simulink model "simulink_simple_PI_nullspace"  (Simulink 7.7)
settings: Solver=ode23t  StartTime=0.0  StopTime=9.6  RelTol=1e-6
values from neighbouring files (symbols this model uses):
  A = [((-UAfr)/mCpf) (UAfr/mCpf) 0; (UAfr/mCpr) ((-UAro-UAfr)/mCpr) 0; 0 0 0]    [simplemodel.m]
  B = [1/mCpf 0 0 ; 0 1/mCpr (UAro/mCpr); 0 1 0]    [simplemodel.m]
  C = [1 0 0; 0 1 0; 0 0 1]    [simplemodel.m]
  D = [0 0 0 ; 0 0 0; 0 0 0]    [simplemodel.m]
  H = [H(:,1) H2 H(:,2) H4 H(:,3) H6 H(:,4)]    [simplemodel.m]
  init = [Tf Tr E]    [simplemodel.m]
  qhf = 0    [simplemodel.m]
  qhr = 4000*60*60    (= 14400000)    [simplemodel.m]
  tc = t1(240)    [simplemodel.m]
  Tc = 293    [simplemodel.m]
  Tc_n = Tc    (= 293)    [simplemodel.m]
  tc_n = tc    [simplemodel.m]
  Tmax = 293    [simplemodel.m]
  Tmin = 283    [simplemodel.m]
  To = 273+0    (= 273)    [simplemodel.m]
  Trset = 293    [simplemodel.m]
  Ts_n = 283    [simplemodel.m]
  ts_n = 3.66    [simplemodel.m]
  ymax = [5  0.4   15    1.44*10^7  0.4396 0.266466 0.1018]'    [simplemodel.m]
  yn = [To_n t_n DeltaT_n qhr_n di_n t_sqrt_n  tsq_n]'    [simplemodel.m]
libraries: simulink x1

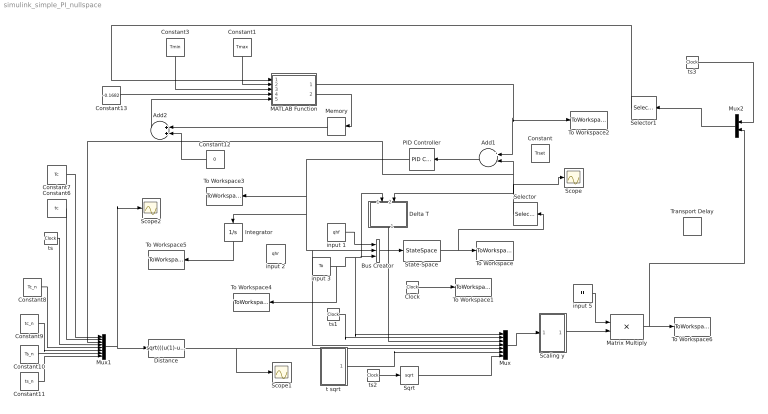
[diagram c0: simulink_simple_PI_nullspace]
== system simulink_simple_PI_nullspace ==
  Add1 : Sum  Inputs=+-
  Add2 : Sum
  Bus Creator : BusCreator  Inputs=3
  Clock : Clock
  Constant : Constant  Value=Trset
  Constant1 : Constant  Value=Tmax
  Constant10 : Constant  Value=Ts_n
  Constant11 : Constant  Value=ts_n
  Constant12 : Constant  Value=0
  Constant13 : Constant  Value=-0.1682
  Constant3 : Constant  Value=Tmin
  Constant6 : Constant  Value=tc
  Constant7 : Constant  Value=Tc
  Constant8 : Constant  Value=Tc_n
  Constant9 : Constant  Value=tc_n
  Delta T : Subsystem
  Distance : Fcn  Expr=sqrt(((u(1)-u(3))/(u(5)-u(7)))^2+((u(2)-u(4))/(u(6)-u(8)))^2)
  Integrator : Integrator
  MATLAB Function : Stateflow chart  TreatAsAtomicUnit=on
  Matrix Multiply : Product  Multiplication=Matrix(*)
  Memory : Memory
  Mux : Mux  Inputs=7
  Mux1 : Mux  Inputs=8
  Mux2 : Mux  Inputs=2
  PID Controller : simulink/Continuous/PID Controller  SystemSampleTime=-1  Controller=PI  TimeDomain=Continuous-time  SampleTime=1  IntegratorMethod=Forward Euler  FilterMethod=Forward Euler  Form=Parallel  P=7032008.284*4  I=175800207.1  D=0  N=100  InitialConditionSource=internal  InitialConditionForIntegrator=0  InitialConditionForFilter=0  ExternalReset=none  LimitOutput=on  UpperSaturationLimit=4000*60*60  LowerSaturationLimit=0  LinearizeAsGain=off  AntiWindupMode=clamping  Kb=1  TrackingMode=off  Kt=1  PParamMin=[]  PParamMax=[]  IParamMin=[]  IParamMax=[]  DParamMin=[]  DParamMax=[]  NParamMin=[]  NParamMax=[]  KbParamMin=[]  KbParamMax=[]  KtParamMin=[]  KtParamMax=[]  POutMin=[]  POutMax=[]  IOutMin=[]  IOutMax=[]  DOutMin=[]  DOutMax=[]  NOutMin=[]  NOutMax=[]  KbOutMin=[]  KbOutMax=[]  KtOutMin=[]  KtOutMax=[]  IntegratorOutMin=[]  IntegratorOutMax=[]  FilterOutMin=[]  FilterOutMax=[]  SumOutMin=[]  SumOutMax=[]  SumI1OutMin=[]  SumI1OutMax=[]  SumI2OutMin=[]  SumI2OutMax=[]  SumI3OutMin=[]  SumI3OutMax=[]  SumDOutMin=[]  SumDOutMax=[]  SaturationOutMin=[]  SaturationOutMax=[]  IntegratorContinuousStateAttributes=''  IntegratorStateMustResolveToSignalObject=off  IntegratorRTWStateStorageClass=Auto  FilterContinuousStateAttributes=''  FilterStateMustResolveToSignalObject=off  FilterRTWStateStorageClass=Auto
  Scaling y : Subsystem
  Scope : Scope
  Scope1 : Scope
  Scope2 : Scope
  Selector : Selector  InputPortWidth=3  IndexOptions=Index vector (dialog)  Indices=2  OutputSizes=1
  Selector1 : Selector  InputPortWidth=3  IndexOptions=Index vector (dialog)  Indices=3  OutputSizes=1
  Sqrt : Sqrt
  State-Space : StateSpace  A=A  B=B  C=C  D=D  X0=init
  To Workspace : ToWorkspace  VariableName=simout_1  SampleTime=-1  SaveFormat=Array
  To Workspace1 : ToWorkspace  VariableName=time_1  SampleTime=-1  SaveFormat=Array
  To Workspace2 : ToWorkspace  VariableName=Set_out_1  SampleTime=-1  SaveFormat=Array
  To Workspace3 : ToWorkspace  VariableName=Qhr  SampleTime=-1  SaveFormat=Array
  To Workspace4 : ToWorkspace  VariableName=To_out  SampleTime=-1  SaveFormat=Array
  To Workspace5 : ToWorkspace  VariableName=E_out_1  SampleTime=-1  SaveFormat=Array
  To Workspace6 : ToWorkspace  VariableName=c  SampleTime=-1  SaveFormat=Array
  Transport Delay : TransportDelay  DelayTime=0.001  InitialOutput=-1
  input 1 : Constant  Value=qhf
  input 2 : Constant  Value=qhr
  input 3 : Constant  Value=To
  input 5 : Constant  Value=H
  t sqrt : Subsystem
  ts{,1..3} (4 alike) : Clock
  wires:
  Bus Creator/1 -> State-Space/1
  State-Space/1 -> To Workspace/1, Selector/1
  Clock/1 -> To Workspace1/1
  Selector/1 -> Scope/1, Delta T/2(In2), Add1/2, Mux1/3
  Add1/1 -> PID Controller/1
  input 1/1 -> Bus Creator/1
  PID Controller/1 -> To Workspace3/1, Bus Creator/2, Mux/4, Integrator/1
  input 3/1 -> To Workspace4/1, Bus Creator/3, Delta T/1(In1), Mux/1
  Integrator/1 -> To Workspace5/1
  Delta T/1(Out1) -> Mux/3
  Matrix Multiply/1 -> To Workspace6/1, Mux2/2
  Scaling y/1(Out1) -> Matrix Multiply/2
  input 5/1 -> Matrix Multiply/1
  ts1/1 -> Mux/2
  Mux1/1 -> Distance/1, Scope2/1
  Constant7/1 -> Mux1/1
  Constant6/1 -> Mux1/2
  ts/1 -> Mux1/4
  Constant8/1 -> Mux1/5
  Constant9/1 -> Mux1/6
  Constant10/1 -> Mux1/7
  Constant11/1 -> Mux1/8
  Distance/1 -> Mux/5, Scope1/1
  Selector1/1 -> MATLAB Function/1(u)
  ts2/1 -> Sqrt/1
  Mux2/1 -> Selector1/1
  ts3/1 -> Mux2/1
  Memory/1 -> Add2/1
  Add2/1 -> MATLAB Function/5(flag)
  Constant1/1 -> MATLAB Function/2(Tmax)
  Constant13/1 -> MATLAB Function/4(ts)
  Constant12/1 -> Add2/2
  MATLAB Function/1(y) -> Add1/1, To Workspace2/1
  MATLAB Function/2(flag1) -> Memory/1
  Constant3/1 -> MATLAB Function/3(Tmin)
  t sqrt/1(Out1) -> Mux/6
  Sqrt/1 -> Mux/7
  Mux/1 -> Scaling y/1(In1)

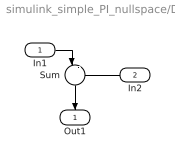
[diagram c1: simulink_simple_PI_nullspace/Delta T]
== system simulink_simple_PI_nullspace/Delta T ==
  In1 : Inport
  In2 : Inport  Port=2
  Sum : Sum  Inputs=|-+
  Out1 : Outport
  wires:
  In1/1 -> Sum/1
  In2/1 -> Sum/2
  Sum/1 -> Out1/1

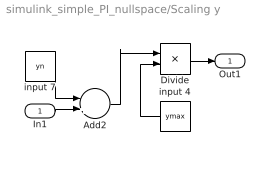
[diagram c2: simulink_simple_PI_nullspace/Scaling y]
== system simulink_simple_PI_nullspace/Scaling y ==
  In1 : Inport
  Add2 : Sum  Inputs=-+
  Divide : Product  Inputs=*/
  input 4 : Constant  Value=ymax
  input 7 : Constant  Value=yn
  Out1 : Outport
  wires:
  input 7/1 -> Add2/1
  input 4/1 -> Divide/2
  Add2/1 -> Divide/1
  Divide/1 -> Out1/1
  In1/1 -> Add2/2

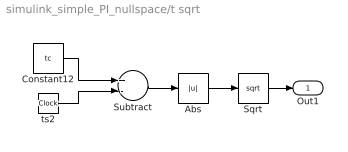
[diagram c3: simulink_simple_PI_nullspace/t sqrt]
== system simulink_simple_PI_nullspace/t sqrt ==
  Abs : Abs
  Constant12 : Constant  Value=tc
  Sqrt : Sqrt
  Subtract : Sum  Inputs=+-
  ts2 : Clock
  Out1 : Outport
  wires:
  Constant12/1 -> Subtract/1
  ts2/1 -> Subtract/2
  Subtract/1 -> Abs/1
  Abs/1 -> Sqrt/1
  Sqrt/1 -> Out1/1

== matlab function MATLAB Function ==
function [y,flag1]= fcn(u,Tmax,Tmin,ts,flag)
%#codegen
if flag==0
if u>=ts
   y=Tmax;
   flag1 = 1;
else 
    y=Tmin;
    flag1 = 0;
end
else
    y=Tmax;
    flag1=1;
end
